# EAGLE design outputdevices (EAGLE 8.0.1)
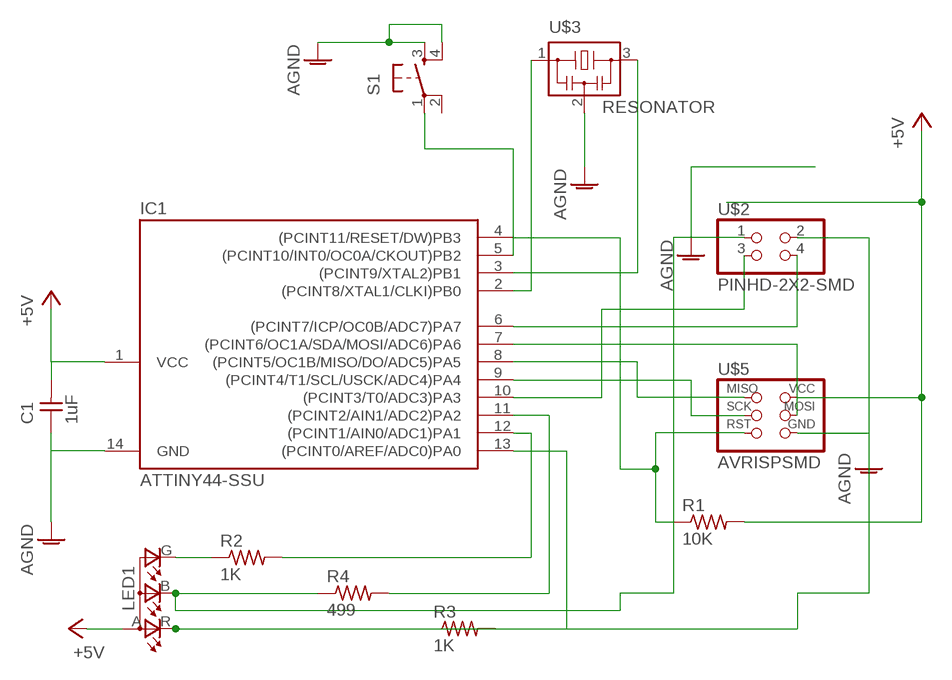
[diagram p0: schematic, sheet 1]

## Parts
C1  1uF  CAP-UNPOLARIZEDFAB  [C1206FAB]
IC1  ATTINY44-SSU  [SOIC14]
LED1  LEDRGBOLD  [P-LCC-4-3]
R1  10K  RES-US1206FAB  [R1206FAB]
R2  1K  RES-US1206FAB  [R1206FAB]
R3  1K  RES-US1206FAB  [R1206FAB]
R4  499  RES-US1206FAB  [R1206FAB]
S1  6MM_SWITCH6MM_SWITCH  [6MM_SWITCH]
U$2  PINHD-2X2-SMD  [2X02SMD]
U$3  RESONATOR  [EFOBM]
U$5  AVRISPSMD  [2X03SMD]

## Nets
+5V: C1.2 IC1.1(VCC) LED1.A(A2) R1.2 U$5.2(VCC)
AGND: C1.1 IC1.14(GND) S1.3(S) S1.4(S1) U$3.2 U$5.6(GND)
N$1: IC1.8((PCINT5/OC1B/MISO/DO/ADC5)PA5) U$5.1(MISO)
N$2: IC1.9((PCINT4/T1/SCL/USCK/ADC4)PA4) U$5.3(SCK)
N$3: IC1.2((PCINT8/XTAL1/CLKI)PB0) U$3.1
N$4: IC1.12((PCINT1/AIN0/ADC1)PA1) R2.2
N$5: IC1.11((PCINT2/AIN1/ADC2)PA2) R4.2
N$6: IC1.13((PCINT0/AREF/ADC0)PA0) R3.2
N$7: IC1.7((PCINT6/OC1A/SDA/MOSI/ADC6)PA6) U$5.4(MOSI)
N$8: IC1.3((PCINT9/XTAL2)PB1) U$3.3
N$9: IC1.4((PCINT11/RESET/DW)PB3) R1.1 U$5.5(RST)
N$10: IC1.10((PCINT3/T0/ADC3)PA3) U$2.3
N$11: IC1.5((PCINT10/INT0/OC0A/CKOUT)PB2) S1.1(P)
N$12: IC1.6((PCINT7/ICP/OC0B/ADC7)PA7) U$2.4
N$13: LED1.G(CGREEN) R2.1
N$15: LED1.R(CRED) R3.1 U$2.2
N$21: LED1.B(CBLUE) R4.1 U$2.1
Unconnected: S1.2(P1)

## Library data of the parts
C1 = fab:CAP-UNPOLARIZED
IC1 = fab:ATTINY44
LED1 = fab:LEDRGBOLD: OSRAM Hyper Multi TOPLED® Hyper-Bright LED LATB T686 Source: http://www.osram.convergy.de/
R1-R4 = fab:RES-US: Resistor (US Symbol)
S1 = fab:6MM_SWITCH: OMRON SWITCH
U$2 = fab:PINHD-2X2-SMD
U$3 = fab:RESONATOR
U$5 = fab:AVRISP

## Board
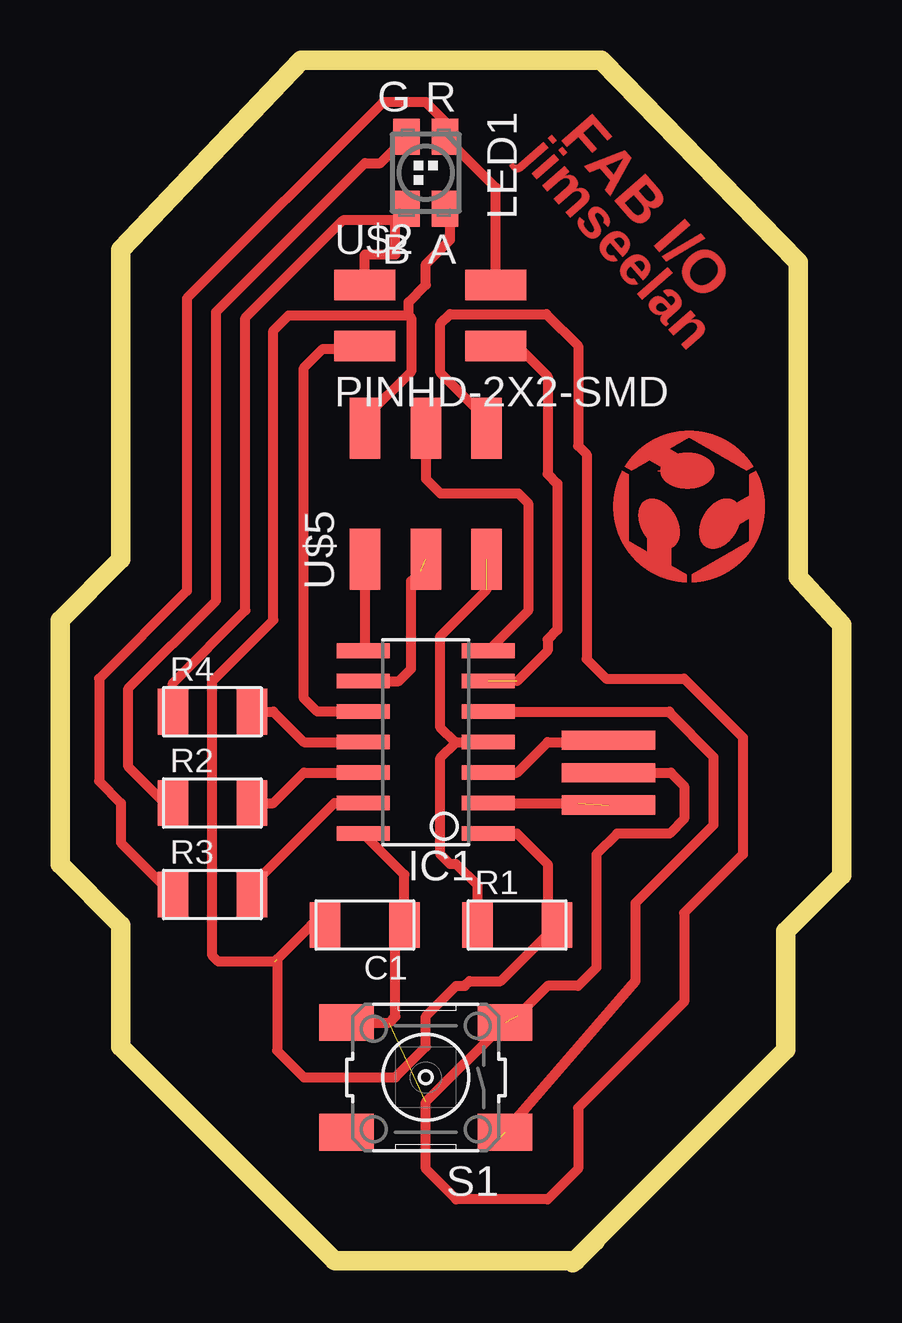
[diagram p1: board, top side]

Size 32.56 x 50.11 mm. Coordinates in mm from the lower left corner, seen from the top.
Outline: 11.43,0.1 2.54,8.99 2.54,14.07 0,16.61 0,26.77 2.54,29.31 2.54,40.74
Outline: 2.54,39.23 2.54,42.21 10.05,50.11 22.55,50.11 30.76,41.68 30.76,28.55 32.56,26.57 32.56,16.13 30.23,13.8 30.23,8.87 21.36,0
Outline: 11.48,0.08 21.49,0.08 22.31,0.9
Copper layers (1*16): Top 0.035mm / dielectric 1.5mm / Bottom 0.035mm
Design rules "default *": minimum track width 16mil, minimum drill 24mil, track to track 16mil, track to pad 16mil, pad to pad 16mil, via to via 16mil, smd to smd 8mil, copper to edge 40mil, drill to drill 8mil, minimum pad ring 10mil, minimum via ring 8mil, stop-mask expansion 4mil, vias tented up to drill 0mil, thermal gap 10mil

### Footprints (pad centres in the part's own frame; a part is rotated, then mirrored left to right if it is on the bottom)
C1206FAB = smd 1.27 x 1.905: 1 -1.651,0; 2 1.651,0
SOIC14 = smd 0.61 x 2.21: 1 -3.81,-2.603; 2 -2.54,-2.603; 3 -1.27,-2.603; 4 0,-2.603; 5 1.27,-2.603; 6 2.54,-2.603; 7 3.81,-2.603; 8 3.81,2.603; 9 2.54,2.603; 10 1.27,2.603; 11 0,2.603; 12 -1.27,2.603; 13 -2.54,2.603; 14 -3.81,2.603
P-LCC-4-3 = smd 1.1 x 1.5: A -0.8,1.5; B 0.8,1.5; G 0.8,-1.5; R -0.8,-1.5
R1206FAB = smd 1.27 x 1.905: 1 -1.651,0; 2 1.651,0
6MM_SWITCH = smd 2.286 x 1.524: 1 -3.302,2.286; 2 3.302,2.286; 3 -3.302,-2.286; 4 3.302,-2.286
2X02SMD = smd 2.54 x 1.27: 1 -2.54,1.27; 2 2.92,1.27; 3 -2.54,-1.27; 4 2.92,-1.27
EFOBM = smd 0.8 x 3.9: 1 -1.35,0; 2 0,0; 3 1.35,0
2X03SMD = smd 2.54 x 1.27: 1 -2.54,2.54; 2 2.92,2.54; 3 -2.54,0; 4 2.92,0; 5 -2.54,-2.54; 6 2.92,-2.54

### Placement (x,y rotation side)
C1  12.7,14.07 180 top
IC1  15.24,21.69 90 top
LED1  15.24,45.41 180 top
R1  19.05,14.07 0 top
R2  6.35,19.15 0 top
R3  6.35,15.34 0 top
R4  6.35,22.96 0 top
S1  15.24,7.72 180 top
U$2  15.24,39.47 0 top
U$3  22.86,20.42 90 top
U$5  15.24,31.85 90 top

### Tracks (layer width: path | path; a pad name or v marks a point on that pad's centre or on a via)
+5V  (1 unrouted)
  Top 0.406: 14.53,39.47 9.53,39.47 8.89,38.83 8.89,26.77 6.35,24.23 6.35,12.8 6.6,12.54 8.94,12.54 10.46,14.07 C1.2 | U$5.2 12.7,35.2 14.63,37.13 14.63,39.36 14.53,39.47 | IC1.1 19.05,17.88 20.32,16.61 20.32,14.45 R1.2 18.36,11.73 17.07,11.73 16.87,11.53 16.51,11.53 15.24,10.26 15.24,8.99 13.97,7.72 10.16,7.72 9.04,8.83 9.04,12.64 | LED1.A 16.26,43.69 16.26,42.62 15.24,41.6 15.24,40.74 14.53,40.03 14.53,39.47
AGND  (2 unrouted)
  Top 0.406: C1.1 14.35,16.16 IC1.14 | C1.1 14.35,13.69 | S1.4 13.72,10 13.97,10.26 13.97,13.69 C1.1 | U$3.2 25.45,20.42 26.01,19.86 26.01,18.49 25.4,17.88 23.22,17.88 22.35,17.01 22.35,12.29 21.59,11.53 20.32,11.53 19.05,10.26 | S1.3 15.24,6.7 15.24,3.91 16.51,2.64 20.32,2.64 21.59,3.91 21.59,6.45 26.01,10.87 26.01,14.57 28.45,17.01 28.45,21.89 26.01,24.33 22.76,24.33 21.95,25.14 21.95,33.68 21.59,34.03 21.59,38.2 20.27,39.52 16.26,39.52 15.85,39.11 15.85,37.08 17.78,35.15 U$5.6 17.4,34.77
N$1
  Top 0.406: U$5.1 12.7,25.56 IC1.8
N$2  (1 unrouted)
  Top 0.406: IC1.9 14.12,24.23 14.63,24.73 14.63,28.39 15.04,28.8
N$3  (1 unrouted)
  Top 0.406: IC1.2 21.59,19.15
N$4
  Top 0.406: R2.2 8.89,19.15 10.16,20.42 IC1.12
N$5
  Top 0.406: R4.2 8.89,22.96 10.16,21.69 IC1.11
N$6
  Top 0.406: R3.2 8,15.72 11.43,19.15 IC1.13
N$7
  Top 0.406: U$5.4 15.24,32.66 15.85,32.05 19.1,32.05 19.51,31.64 19.51,27.16 IC1.7
N$8
  Top 0.406: IC1.3 19.05,20.42 20.32,21.69 22.78,21.69 U$3.3
N$9  (1 unrouted)
  Top 0.406: 16.51,21.69 15.85,21.03 15.85,17.01 16.26,16.61 16.51,16.61 17.4,15.72 R1.1 | 16.51,21.69 IC1.4 | 16.51,21.69 16.46,21.69 15.85,22.3 15.85,26.11 17.78,28.04
N$10
  Top 0.406: IC1.10 10.72,22.96 10.16,23.52 10.16,37.28 10.95,38.07 12.58,38.07 U$2.3
N$11  (1 unrouted)
  Top 0.406: IC1.5 25.4,22.96 25.4,22.91 27.23,21.08 27.23,18.23 23.98,14.98 23.98,11.73 18.37,5.25
N$12  (1 unrouted)
  Top 0.406: U$2.4 19.05,38.2 20.32,36.93 20.32,32.86 20.73,32.46 20.73,26.36 20.32,25.95 20.32,25.5 19.05,24.23
N$13
  Top 0.406: R2.1 4.37,19.15 2.84,20.67 2.84,23.92 6.5,27.58 6.5,39.62 12.7,45.82 13.35,45.82 LED1.G
N$15
  Top 0.406: R3.1 2.54,17.5 2.54,19.15 1.63,20.06 1.63,24.33 5.28,27.99 5.28,40.18 13.46,48.36 15.24,48.36 16.04,47.56 LED1.R 18.16,44.79 U$2.2
N$21
  Top 0.406: R4.1 4.7,24.15 7.72,27.17 7.72,39.36 11.79,43.43 13.96,43.43 | 13.96,43.43 LED1.B | U$2.1 12.7,42.01 13.97,42.01 13.97,43.42 13.96,43.43
(copper drawn outside any net)
  shapes: Top area x3419

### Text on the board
Top: FAB I/O | jimseelan | E:/EagleFiles/logo.bmp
